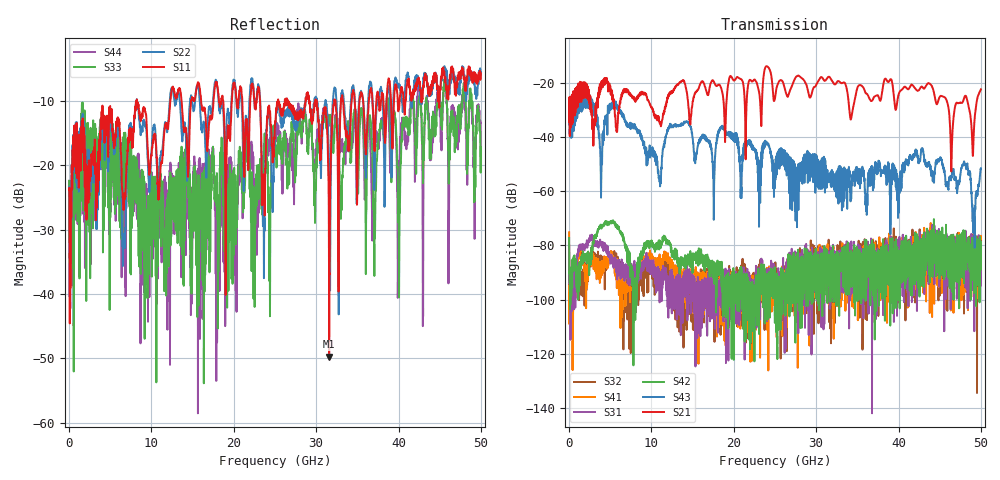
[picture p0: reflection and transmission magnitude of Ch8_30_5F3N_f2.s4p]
!Agilent Technologies,N5247A,US51170199,A.09.90.13
!Agilent N5247A: A.09.90.13
!Date: Wednesday, December 16, 2015 10:32:37
!Correction: S11(Full 4 Port(1,2,3,4))
!S12(Full 4 Port(1,2,3,4))
!S13(Full 4 Port(1,2,3,4))
!S14(Full 4 Port(1,2,3,4))
!S21(Full 4 Port(1,2,3,4))
!S22(Full 4 Port(1,2,3,4))
!S23(Full 4 Port(1,2,3,4))
!S24(Full 4 Port(1,2,3,4))
!S31(Full 4 Port(1,2,3,4))
!S32(Full 4 Port(1,2,3,4))
!S33(Full 4 Port(1,2,3,4))
!S34(Full 4 Port(1,2,3,4))
!S41(Full 4 Port(1,2,3,4))
!S42(Full 4 Port(1,2,3,4))
!S43(Full 4 Port(1,2,3,4))
!S44(Full 4 Port(1,2,3,4))
!S4P File: Measurements: <S11,S12,S13,S14>,
!<S21,S22,S23,S24>,
!<S31,S32,S33,S34>,
!<S41,S42,S43,S44>:
# Hz S  dB  R 50
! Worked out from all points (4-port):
!   3201 points, 10 MHz to 50 GHz, reference 50 ohm
!   strongest paths, dB at 10 MHz, 12.51 GHz, 25 GHz, 37.5 GHz, 50 GHz:
!     S21: -34.4, -23.5, -25.6, -24.6, -22.3
!     S43: -35.3, -36.1, -49.8, -50.1, -51.5
!     S42: -77.3, -82.7, -92.6, -84.5, -78.5
!     S31: -80.1, -104.1, -90.1, -91.0, -94.9
!     S41: -75.2, -92.5, -92.0, -92.4, -78.3
!     S32: -84.8, -99.6, -88.5, -101.2, -88.6
!   lowest |S11| = -49.8 dB at 31.58 GHz (marker M1), VSWR 1.01, Z = 50.2 + j0.218 ohm
!   |S11| at or under -10 dB: start of sweep to 8.215 GHz; 8.25 GHz to 12.28 GHz (4.032 GHz wide, 39.3 % of centre); 23.2 GHz to 25.35 GHz (2.159 GHz wide, 8.89 % of centre)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
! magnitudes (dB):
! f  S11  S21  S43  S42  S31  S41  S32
! 10 MHz  -23.8  -34.4  -35.3  -77.3  -80.1  -75.2  -84.8
! 15.66 GHz  -7.1  -22.3  -43.0  -82.0  -99.6  -93.8  -91.0
! 31.58 GHz  -49.8  -17.7  -54.3  -87.8  -86.1  -84.2  -97.2
! 43.77 GHz  -8.5  -20.1  -50.6  -91.0  -85.9  -83.1  -82.9
! 46.44 GHz  -5.5  -49.2  -54.4  -79.3  -82.5  -91.9  -83.8
! 49.14 GHz  -6.9  -38.1  -70.7  -86.5  -87.6  -78.3  -87.3
! 50 GHz  -5.7  -22.3  -51.5  -78.5  -94.9  -78.3  -88.6
